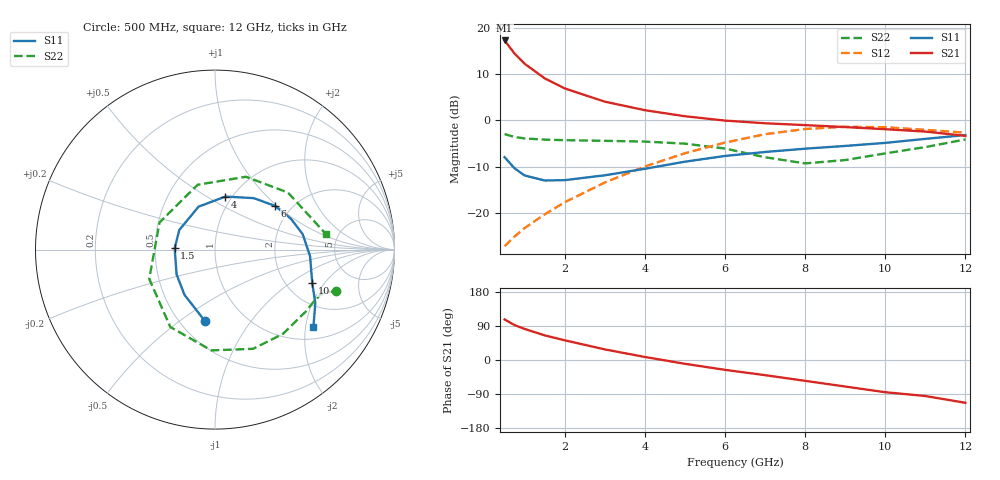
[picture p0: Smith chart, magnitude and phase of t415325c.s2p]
!AT-41532
!S-PARAMETERS at Vce=5V  Ic=5mA.  LAST UPDATED 05-29-98
# ghz s ma r 50
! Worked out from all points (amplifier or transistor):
!   15 points, 500 MHz to 12 GHz, reference 50 ohm
!   highest |S21| = 17.3 dB at 500 MHz (marker M1)
!   |S21| within 3 dB of that: start of sweep to 767.2 MHz
!   unconditionally stable (mu >= 1): 992.5 MHz to 2.182 GHz
!   at 1 GHz: K = 1.00, MAG = 17.4 dB, |S12| = -23.2 dB
!   at 5 GHz: K = 0.76, MSG = 4.0 dB, |S12| = -7.1 dB
!   at 12 GHz: K = 0.99, MSG = -0.3 dB, |S12| = -2.6 dB
!   lowest NFmin = 1.10 dB at 900 MHz
!   S11 on the Smith chart (normalised r, x): 500 MHz: 0.66, -0.63; 1.5 GHz: 0.63, +0.01; 4 GHz: 0.93, +0.61; 6 GHz: 1.65, +0.97; 10 GHz: 2.74, -1.52; 12 GHz: 1.33, -2.21
0.5  0.402 -98.0  7.303 107.0  0.044 60.0  0.713 -19.0
0.75  0.304 -124.0  5.26 92.0  0.056 61.0  0.663 -21.0
1  0.255 -147.0  4.095 82.0  0.069 63.0  0.64 -23.0
1.5  0.225 178.0  2.848 65.0  0.097 66.0  0.621 -28.0
2  0.227 151.0  2.218 52.0  0.131 65.0  0.613 -34.0
3  0.256 111.0  1.596 28.0  0.214 59.0  0.603 -51.0
4  0.301 79.0  1.291 8.0  0.319 48.0  0.592 -69.0
5  0.359 53.0  1.111 -10.0  0.443 33.0  0.562 -92.0
6  0.414 36.0  0.997 -26.0  0.577 16.0  0.498 -120.0
7  0.457 22.0  0.933 -40.0  0.711 -4.0  0.401 -156.0
8  0.496 10.0  0.891 -55.0  0.809 -26.0  0.344 154.0
9  0.531 -4.0  0.849 -70.0  0.854 -49.0  0.374 105.0
10  0.573 -19.0  0.805 -85.0  0.847 -69.0  0.441 67.0
11  0.633 -28.0  0.759 -95.0  0.792 -88.0  0.516 38.0
12  0.696 -38.0  0.682 -113.0  0.739 -105.0  0.624 8.0
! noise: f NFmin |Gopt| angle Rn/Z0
0.9  1.1  0.29  110  0.14
1.8  1.4  0.41  -167  0.08
2  1.5  0.44  -153  0.09
2.5  1.7  0.53  -127  0.19
3  1.9  0.6  -106  0.37
3.5  2.2  0.67  -86  0.74
4  2.4  0.71  -70  1.19
